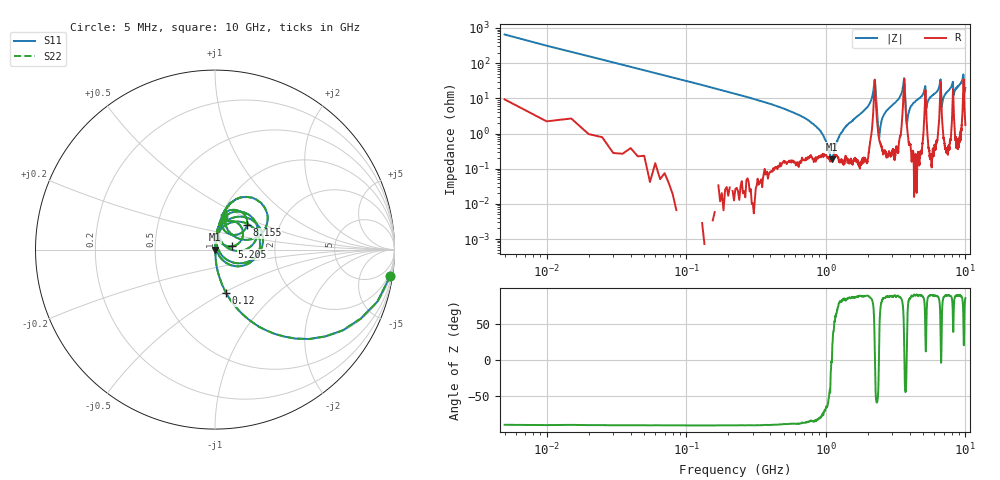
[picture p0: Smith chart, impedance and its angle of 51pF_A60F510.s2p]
! Amotech Co.,Ltd.
! http://www.amotech.co.kr/
! Part Number: A60F510
! These Parameters are Measured in Series Mode Connection
! Operation Temp=25[degC], DC Bias Voltage=0[V]
! Freq. Start=5[MHz] Stop=10[GHz], 2000[Steps]
! Date: Monday, July 20, 2020, 04:25:20
# GHZ S RI R 50.000000
!Freq.(Hz) S11(Real) S11(Imag) S21(Real) S21(Imag) S12(Real) S12(Imag) S22(Real) S22(Imag)
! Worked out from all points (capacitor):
!   2000 points, 5 MHz to 10 GHz, reference 50 ohm
!   read as one part in series: C = 50.5 pF near 55 MHz
!   lowest |Z| = 184 mohm at 1.105 GHz (marker M1)
!   series resonance near 1.106 GHz, so ESL is about 410 pH
!   S11 on the Smith chart (normalised r, x): 5 MHz: 1, -13; 120 MHz: 1.00, -0.52; 5.205 GHz: 1.21, +0.04; 8.155 GHz: 1.37, +0.39; 10 GHz: 1.03, +0.40
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0.005  0.9751 -0.1489  0.0249 0.1489  0.0249 0.1489  0.9751 -0.1489
0.12  0.063 -0.2432  0.937 0.2432  0.937 0.2432  0.063 -0.2432
0.875  0.00222 -0.0139  0.9978 0.0139  0.9978 0.0139  0.00222 -0.0139
1.105  0.00184 -0.000103  0.9982 0.000103  0.9982 0.000103  0.00184 -0.000103
1.31  0.00184 0.0109  0.9982 -0.0109  0.9982 -0.0109  0.00184 0.0109
1.675  0.00269 0.0303  0.9973 -0.0303  0.9973 -0.0303  0.00269 0.0303
2.23  0.212 0.1228  0.788 -0.1228  0.788 -0.1228  0.212 0.1228
2.42  0.00623 0.00495  0.9938 -0.00495  0.9938 -0.00495  0.00623 0.00495
2.655  0.0048 0.0379  0.9952 -0.0379  0.9952 -0.0379  0.0048 0.0379
3.34  0.0151 0.0961  0.9849 -0.0961  0.9849 -0.0961  0.0151 0.0961
3.635  0.2591 0.1019  0.7409 -0.1019  0.7409 -0.1019  0.2591 0.1019
3.82  0.015 0.0114  0.985 -0.0114  0.985 -0.0114  0.015 0.0114
4.07  0.00673 0.0588  0.9933 -0.0588  0.9933 -0.0588  0.00673 0.0588
5.005  0.0283 0.134  0.9717 -0.134  0.9717 -0.134  0.0283 0.134
5.205  0.0942 0.0176  0.9058 -0.0176  0.9058 -0.0176  0.0942 0.0176
6.67  0.1956 0.0145  0.8044 -0.0145  0.8044 -0.0145  0.1956 0.0145
6.78  0.0351 0.0444  0.9649 -0.0444  0.9649 -0.0444  0.0351 0.0444
8.155  0.1777 0.1355  0.8223 -0.1355  0.8223 -0.1355  0.1777 0.1355
8.335  0.0384 0.1405  0.9616 -0.1405  0.9616 -0.1405  0.0384 0.1405
9.635  0.2343 0.2763  0.7657 -0.2763  0.7657 -0.2763  0.2343 0.2763
9.81  0.0864 0.0908  0.9136 -0.0908  0.9136 -0.0908  0.0864 0.0908
10  0.0529 0.1842  0.9471 -0.1842  0.9471 -0.1842  0.0529 0.1842
